(* Logix 5000 AddOnInstructionDefinition export AOI_ISC_InDataConversion; software revision 32.02 *)

ADD_ON_INSTRUCTION AOI_ISC_InDataConversion   (* revision 1.0 *)
// Input data conversions for ISC CAM IDL V2.0
VAR_INPUT
   InputWord4 : INT; {required}   // Input Word 4 Data Mapping for Communication
   InputWord6 : INT; {required}   // Input Word 6 Data Mapping for Communication
   InputWord12 : INT; {required}   // Input Word 12 Data Mapping for Communication
        .8   // Parameter Read OK
        .9   // Parameter Write OK
        .10   // Parameter Type OK
        .11   // Parameter Value OK
END_VAR
VAR_OUTPUT
   ProductsOnBelt : INT; {access Read Only, required}   // Number of Products on the Belt
   BeltSpeed : INT; {access Read Only, required}
   LastProductDest : INT; {access Read Only, required}   // Last Product Destination
   ParameterGroup : INT; {access Read Only, required}   // Parameter Group
   ParameterReadOK : BOOL; {access None, required}   // Parameter Read OK
   ParameterTypeOK : BOOL; {access None, required}   // Parameter Type OK
   ParameterValueOK : BOOL; {access None, required}   // Parameter Value Format OK
   ParameterWriteOK : BOOL; {access None, required}   // Parameter Write OK
END_VAR
VAR
   BTDT_IW4B0 : FBD_BIT_FIELD_DISTRIBUTE := (Length := 1); {access None}
   BTDT_IW6B0 : FBD_BIT_FIELD_DISTRIBUTE := (Length := 1); {access None}
   BTDT_IW12B0 : FBD_BIT_FIELD_DISTRIBUTE := (Length := 1); {access None}
   BTDT_IW4B1 : FBD_BIT_FIELD_DISTRIBUTE := (Length := 1); {access None}
END_VAR

ROUTINE Logic   (* structured text *)
   //Input Word 4 Mapping
   BTDT_IW4B0.Source:=InputWord4;
   BTDT_IW4B0.SourceBit:=0;
   BTDT_IW4B0.DestBit:=0;
   BTDT_IW4B0.Length:=8;
   BTDT_IW4B0.Target:=ProductsOnBelt;
   BTDT(BTDT_IW4B0);
   ProductsOnBelt:=BTDT_IW4B0.Dest;
   
   BTDT_IW4B1.Source:=InputWord4;
   BTDT_IW4B1.SourceBit:=8;
   BTDT_IW4B1.DestBit:=0;
   BTDT_IW4B1.Length:=8;
   BTDT_IW4B1.Target:=BeltSpeed;
   BTDT(BTDT_IW4B1);
   BeltSpeed:=BTDT_IW4B1.Dest;
   
   //Input Word 6 Mapping
   BTDT_IW6B0.Source:=InputWord6;
   BTDT_IW6B0.SourceBit:=0;
   BTDT_IW6B0.DestBit:=0;
   BTDT_IW6B0.Length:=8;
   BTDT_IW6B0.Target:=LastProductDest;
   BTDT(BTDT_IW6B0);
   LastProductDest:=BTDT_IW6B0.Dest;
   
   //Input Word 12 Mapping
   BTDT_IW12B0.Source:=InputWord12;
   BTDT_IW12B0.SourceBit:=0;
   BTDT_IW12B0.DestBit:=0;
   BTDT_IW12B0.Length:=8;
   BTDT_IW12B0.Target:=ParameterGroup;
   BTDT(BTDT_IW12B0);
   ParameterGroup:=BTDT_IW12B0.Dest;
   
   ParameterReadOK:=InputWord12.8;
   ParameterWriteOK:=InputWord12.9;
   ParameterTypeOK:=InputWord12.10;
   ParameterValueOK:=InputWord12.11;
END_ROUTINE
END_ADD_ON_INSTRUCTION
